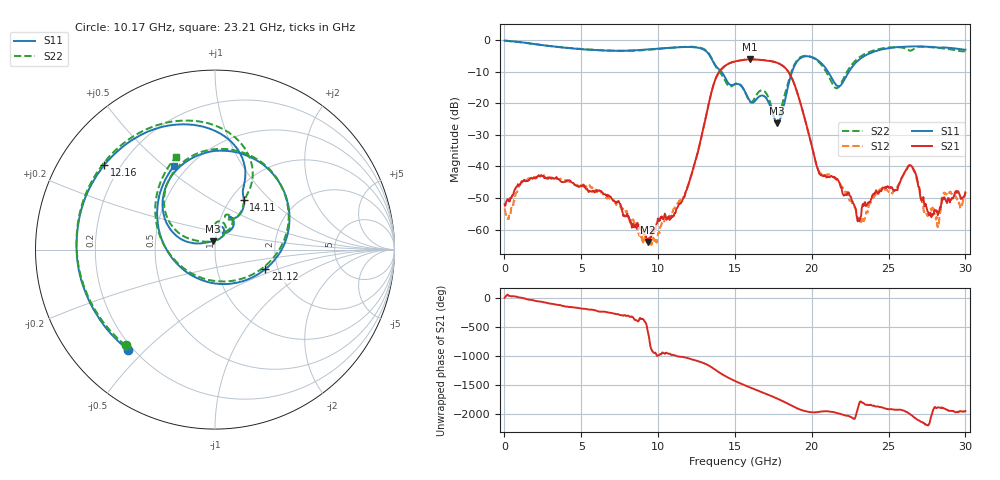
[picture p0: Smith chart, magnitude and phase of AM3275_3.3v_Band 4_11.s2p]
!Keysight Technologies,N5245B,MY58422270,A.16.20.02
!Date: Thursday, March 27, 2025 02:09:04
!Correction: S11(C  2-Port  )
!S21(C  2-Port  )
!S12(C  2-Port  )
!S22(C  2-Port  )
!S2P File: Measurements: S11, S21, S12, S22:
# Hz S  dB  R 50
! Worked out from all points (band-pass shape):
!   801 points, 10 MHz to 30 GHz, reference 50 ohm
!   highest |S21| = -6.09 dB at 15.98 GHz (marker M1); lowest = -63.9 dB at 9.344 GHz (marker M2)
!   |S21| within 3 dB of the highest: 14.14 GHz to 18.33 GHz (4.186 GHz wide, 25.8 % of centre)
!   lowest |S11| = -26.3 dB at 17.74 GHz (marker M3), VSWR 1.10, Z = 48.7 + j4.6 ohm
!   |S11| at or under -10 dB: 14.12 GHz to 18.72 GHz (4.603 GHz wide, 28 % of centre); 21.06 GHz to 22.42 GHz (1.361 GHz wide, 6.26 % of centre)
!   |S22| runs from -26.1 to -0.1 dB; largest |S21 - S12| = 0.0045
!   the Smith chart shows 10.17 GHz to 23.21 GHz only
!   S11 on the Smith chart (normalised r, x): 10.17 GHz: 0.18, -0.44; 12.16 GHz: 0.14, +0.33; 14.11 GHz: 1.15, +0.71; 21.12 GHz: 1.71, -0.41; 23.21 GHz: 0.42, +0.54
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1e7  -0.17 -4.1  -52.01 4.9  -53.36 -117.0  -0.11 -4.6
1.2096e9  -0.74 -80.9  -44.73 -1.0  -44.44 -7.1  -0.78 -81.1
2.596638e9  -1.67 -158.7  -43.66 -75.2  -42.84 -78.5  -1.68 -159.1
5.033325e9  -2.90 92.4  -46.29 177.8  -46.00 178.2  -2.80 91.5
7.2076e9  -3.39 0.6  -51.21 86.2  -51.55 93.0  -3.38 -1.1
9.344388e9  -2.98 -94.6  -63.94 127.2  -64.08 42.3  -3.08 -96.9
1.001916e10  -2.72 -124.3  -57.15 95.4  -61.25 165.1  -2.80 -126.6
1.016911e10  -2.64 -130.9  -56.00 111.3  -58.96 137.2  -2.73 -133.0
1.215595e10  -2.20 142.6  -42.70 26.3  -43.12 28.9  -2.10 140.9
1.41053e10  -9.91 59.8  -9.30 137.7  -9.28 137.7  -10.74 57.3
1.5005e10  -14.00 66.7  -6.76 11.6  -6.76 11.6  -13.86 72.6
1.597968e10  -19.34 59.4  -6.09 -98.9  -6.08 -99.0  -19.58 68.8
1.68044e10  -17.56 72.9  -6.32 173.9  -6.32 173.9  -15.92 76.7
1.774159e10  -26.33 102.6  -7.17 70.7  -7.18 70.7  -25.97 111.3
1.894119e10  -7.57 133.3  -14.94 -86.1  -14.96 -86.1  -7.14 128.6
2.002832e10  -5.42 55.3  -33.93 -166.8  -34.13 -169.5  -5.47 52.0
2.111546e10  -10.44 -21.4  -43.30 -153.1  -42.50 -150.3  -11.64 -29.1
2.321476e10  -5.70 116.2  -55.67 15.7  -57.69 19.2  -5.06 113.0
2.501416e10  -2.57 52.2  -46.79 -114.9  -48.09 -117.7  -2.34 49.8
2.647618e10  -2.00 11.2  -39.77 144.4  -39.57 149.4  -3.29 12.9
2.745085e10  -2.04 -16.4  -52.66 -21.9  -55.05 -16.0  -2.16 -16.0
3e10  -3.05 -107.0  -48.36 -144.2  -47.92 -132.6  -3.55 -108.6
